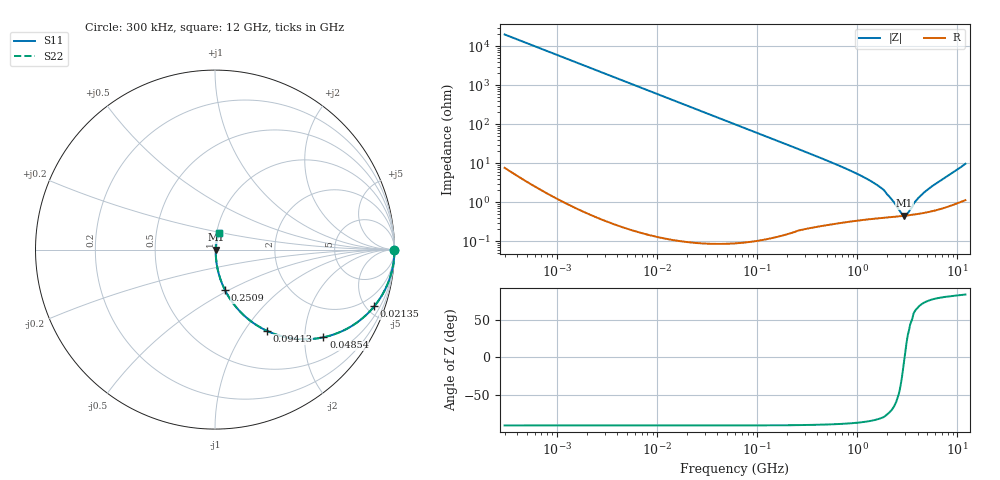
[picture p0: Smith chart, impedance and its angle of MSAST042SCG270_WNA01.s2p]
! MSAST042SCG270_WNA01  S-PARAMETER MODEL  ( General Type )
! Model Generated by TAIYO YUDEN Corporation (http://www.ty-top.com)
! Version 1.0
! TAIYO YUDEN Control No. 150820
! Copyright(c) 2015 TAIYO YUDEN CO.,LTD. All Rights Reserved.
! Product Description (link to TY-COMPAS)
! https://ds.yuden.co.jp/TYCOMPAS/or/detail?pn=MSAST042SCG270JWNA01&u=M
! Products Name : Multilayer Ceramic Capacitors
! Characteristics :
!  Capacitance : 27 pF , Rated Voltage : 25V , TCC : CG / C0G
!  Case Size : 0.4 x 0.2 / 0.016 x 0.008 [mm/inch] , Thickness : 0.2 / 0.008 [mm/inch]
!  (Conditions: Temperature = 25 degC , DC Bias Current/Voltage = 0A / 0V)
! External Node Assignments :
!  1  o---| |---o  2
! GND o---------o GND
! Frequency Range : 0.3MHz  -  12000MHz  [ 401 STEP ]
# MHz S RI R 50
! Freq[MHz].  S11 Real  S11 Imag  S21 Real  S21 Imag  S12 Real  S12 Imag  S22 Real  S22 Imag
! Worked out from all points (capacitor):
!   401 points, 300 kHz to 12 GHz, reference 50 ohm
!   read as one part in series: C = 26.6 pF near 316.3 kHz
!   lowest |Z| = 450 mohm at 2.947 GHz (marker M1)
!   series resonance near 2.966 GHz, so ESL is about 110 pH
!   S11 on the Smith chart (normalised r, x): 300 kHz: open; 21.35 MHz: 1.00, -5.61; 48.54 MHz: 1.00, -2.47; 94.13 MHz: 1.00, -1.27; 250.9 MHz: 1.00, -0.47; 12 GHz: 1.02, +0.19
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0.3  1 -0.005  2.7e-05 0.005  2.7e-05 0.005  1 -0.005
1.769972  0.9991 -0.0295  0.000876 0.0295  0.000876 0.0295  0.9991 -0.0295
4.84353  0.9935 -0.0803  0.0065 0.0803  0.0065 0.0803  0.9935 -0.0803
10.44266  0.9705 -0.1691  0.0295 0.1691  0.0295 0.1691  0.9705 -0.1691
21.35258  0.8873 -0.3161  0.1127 0.3161  0.1127 0.3161  0.8873 -0.3161
31.77076  0.7805 -0.4137  0.2195 0.4137  0.2195 0.4137  0.7805 -0.4137
48.54115  0.6037 -0.4888  0.3963 0.4888  0.3963 0.4888  0.6037 -0.4888
60  0.4993 -0.4996  0.5007 0.4996  0.5007 0.4996  0.4993 -0.4996
94.13233  0.2884 -0.4522  0.7116 0.4522  0.7116 0.4522  0.2884 -0.4522
147.6816  0.1416 -0.3471  0.8584 0.3471  0.8584 0.3471  0.1416 -0.3471
250.8588  0.0548 -0.2238  0.9452 0.2238  0.9452 0.2238  0.0548 -0.2238
353.9943  0.0292 -0.1617  0.9708 0.1617  0.9708 0.1617  0.0292 -0.1617
743.2595  0.00866 -0.0747  0.9913 0.0747  0.9913 0.0747  0.00866 -0.0747
1229.528  0.0052 -0.0401  0.9948 0.0401  0.9948 0.0401  0.0052 -0.0401
1735.023  0.00444 -0.0226  0.9956 0.0226  0.9956 0.0226  0.00444 -0.0226
2088.533  0.00428 -0.0132  0.9957 0.0132  0.9957 0.0132  0.00428 -0.0132
2722.03  0.00439 -0.00304  0.9956 0.00304  0.9956 0.00304  0.00439 -0.00304
2947.191  0.00448 -0.000189  0.9955 0.000189  0.9955 0.000189  0.00448 -0.000189
3190.978  0.00459 0.00261  0.9954 -0.00261  0.9954 -0.00261  0.00459 0.00261
3841.137  0.00498 0.00963  0.995 -0.00963  0.995 -0.00963  0.00498 0.00963
4875.354  0.00578 0.0187  0.9942 -0.0187  0.9942 -0.0187  0.00578 0.0187
12000  0.0201 0.0932  0.9799 -0.0932  0.9799 -0.0932  0.0201 0.0932
